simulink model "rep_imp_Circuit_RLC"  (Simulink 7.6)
settings: Solver=ode23t  StartTime=0.0  StopTime=0.02  RelTol=1e-3
InitFcn:
  | clc
StopFcn:
  | close all
  | load Ie_Vs.mat
  | plot(x(1,:),x(2,:))
  | hold on
  | plot(x(1,:),x(3,:))
  | axis([0 0.02 -0.2 1.20])
  | grid
  | title('Courant d''entrée et tension de sortie')
  | xlabel('temps')
libraries: powerlib x11

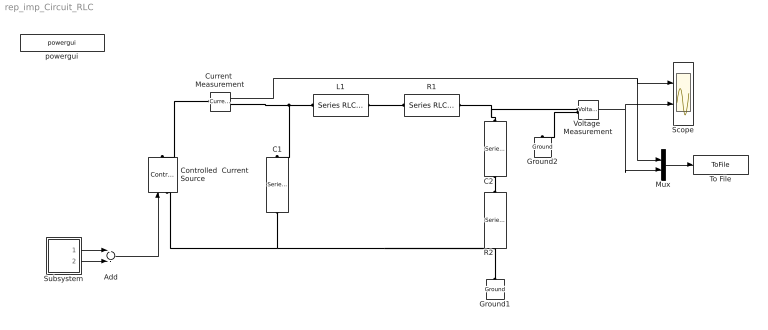
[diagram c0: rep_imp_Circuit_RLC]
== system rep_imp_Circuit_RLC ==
  Add : Sum  Inputs=+-
  C1 : powerlib/Elements/Series RLC Branch  DialogController=POWERSYS.PowerSysDialog  PhysicalDomain=powersysdomain  SubClassName=unknown  LeftPortType=p1  RightPortType=p1  LConnTagsString=__new0  RConnTagsString=__new0  BranchType=C  Resistance=1  Inductance=1e-3  SetiL0=off  InitialCurrent=0  Capacitance=0.001  Setx0=off  InitialVoltage=0  Measurements=None
  C2 : powerlib/Elements/Series RLC Branch  DialogController=POWERSYS.PowerSysDialog  PhysicalDomain=powersysdomain  SubClassName=unknown  LeftPortType=p1  RightPortType=p1  LConnTagsString=__new0  RConnTagsString=__new0  BranchType=C  Resistance=1  Inductance=1e-3  SetiL0=off  InitialCurrent=0  Capacitance=0.001  Setx0=off  InitialVoltage=0  Measurements=None
  Controlled  Current Source : powerlib/Electrical Sources/Controlled Current Source  DialogController=POWERSYS.PowerSysDialog  SystemSampleTime=-1  Initialize=on  Source_Type=AC  Amplitude=0  Phase=0  Frequency=0  Measurements=None
  Current  Measurement : powerlib/Measurements/Current Measurement  DialogController=POWERSYS.PowerSysDialog  SystemSampleTime=-1  PhasorSimulation=off  OutputType=Complex  PSBequivalent=0
  Ground1 : powerlib/Elements/Ground  DialogController=POWERSYS.PowerSysDialog  PhysicalDomain=powersysdomain  SubClassName=unknown  LeftPortType=p1  RightPortType=p1  LConnTagsString=a
  Ground2 : powerlib/Elements/Ground  DialogController=POWERSYS.PowerSysDialog  PhysicalDomain=powersysdomain  SubClassName=unknown  LeftPortType=p1  RightPortType=p1  LConnTagsString=a
  L1 : powerlib/Elements/Series RLC Branch  DialogController=POWERSYS.PowerSysDialog  PhysicalDomain=powersysdomain  SubClassName=unknown  LeftPortType=p1  RightPortType=p1  LConnTagsString=__new0  RConnTagsString=__new0  BranchType=L  Resistance=4  Inductance=1e-3  SetiL0=off  InitialCurrent=0  Capacitance=0  Setx0=off  InitialVoltage=0  Measurements=None
  Mux : Mux  Inputs=2
  R1 : powerlib/Elements/Series RLC Branch  DialogController=POWERSYS.PowerSysDialog  PhysicalDomain=powersysdomain  SubClassName=unknown  LeftPortType=p1  RightPortType=p1  LConnTagsString=__new0  RConnTagsString=__new0  BranchType=R  Resistance=1  Inductance=10e-3  SetiL0=off  InitialCurrent=0  Capacitance=0  Setx0=off  InitialVoltage=0  Measurements=None
  R2 : powerlib/Elements/Series RLC Branch  DialogController=POWERSYS.PowerSysDialog  PhysicalDomain=powersysdomain  SubClassName=unknown  LeftPortType=p1  RightPortType=p1  LConnTagsString=__new0  RConnTagsString=__new0  BranchType=R  Resistance=1  Inductance=10e-3  SetiL0=off  InitialCurrent=0  Capacitance=0  Setx0=off  InitialVoltage=0  Measurements=None
  Scope : Scope  NumInputPorts=2
  Subsystem : Subsystem
  To File : ToFile  Filename=Ie_Vs  MatrixName=x
  Voltage  Measurement : powerlib/Measurements/Voltage Measurement  DialogController=POWERSYS.PowerSysDialog  SystemSampleTime=-1  PhasorSimulation=off  OutputType=Complex  PSBequivalent=0
  powergui : powerlib/powergui  Priority=1  SystemSampleTime=-1  SimulationMode=Continuous  SampleTime=50e-6  frequency=60  SPID=off  DisableSnubberDevices=off  DisableRonSwitches=off  DisableVfSwitches=off  SwTol=0  Interpol=off  frequencyindice=0  echomessages=off  HookPort=off  DisplayEquations=off  FunctionMessages=off  EnableUseOfTLC=off  x0status=blocks  RestoreLinks=warning  ResistiveCurrentMeasurement=off  Frange=[0:2:500]  Ylog=off  Xlog=on  ShowGrid=on  save=off  variable=ZData  ZoomFFT=off  StartTime=0.0  cycles=1  DisplayStyle=1  fundamental=60  FreqAxis=off  MaxFrequency=1000  frequencyindicesteady=1  display=off  methode=off
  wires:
  Voltage  Measurement/1 -> Scope/2, Mux/2
  Subsystem/1(step1) -> Add/1
  Subsystem/2(step2) -> Add/2
  Add/1 -> Controlled  Current Source/1
  Current  Measurement/1 -> Scope/1, Mux/1
  Mux/1 -> To File/1
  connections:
  C1/RConn1 -- R2/LConn1 -- Ground1/LConn1 -- Controlled  Current Source/LConn1
  Voltage  Measurement/LConn2 -- Ground2/LConn1
  C2/LConn1 -- R1/RConn1 -- Voltage  Measurement/LConn1
  R1/LConn1 -- L1/RConn1
  C2/RConn1 -- R2/RConn1
  L1/LConn1 -- C1/LConn1 -- Current  Measurement/RConn1
  Current  Measurement/LConn1 -- Controlled  Current Source/RConn1

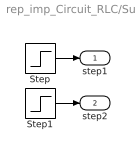
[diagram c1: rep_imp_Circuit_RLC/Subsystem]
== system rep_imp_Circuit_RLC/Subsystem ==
  Step : Step  Time=0.004  SampleTime=0
  Step1 : Step  Time=0.006  SampleTime=0
  step1 : Outport
  step2 : Outport  Port=2
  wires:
  Step/1 -> step1/1
  Step1/1 -> step2/1
